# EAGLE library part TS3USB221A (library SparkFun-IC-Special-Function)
DPDT Analog Mux DPDT Analog Mux Vcc 2.5 to 3.3V Passes up to 5.5V at 3.3V supply 900MHz BW, 6&#8486; switch resistance SparkFun Products SparkFun FTDI SmartBasic (DEV-12935)
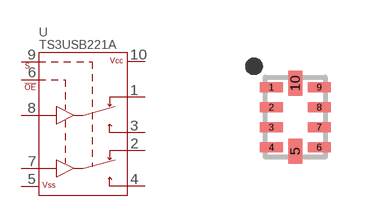
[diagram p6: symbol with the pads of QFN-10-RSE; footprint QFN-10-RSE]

Designator prefix U

## TS3USB221A (PROD_ID: IC-12115; VALUE: TS3USB221A)  [QFN-10-RSE]
1  1D+
2  1D-
3  2D+
4  2D-
5  VSS
6  !OE
7  D-
8  D+
9  S
10  VCC

## Footprint QFN-10-RSE (pad centres in mm)
smd 0.58 x 0.25: 1 -0.6,0.75; 2 -0.6,0.25; 3 -0.6,-0.25; 4 -0.6,-0.75; 6 0.6,-0.75; 7 0.6,-0.25; 8 0.6,0.25; 9 0.6,0.75
smd 0.35 x 0.63: 5 0,-0.85; 10 0,0.85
